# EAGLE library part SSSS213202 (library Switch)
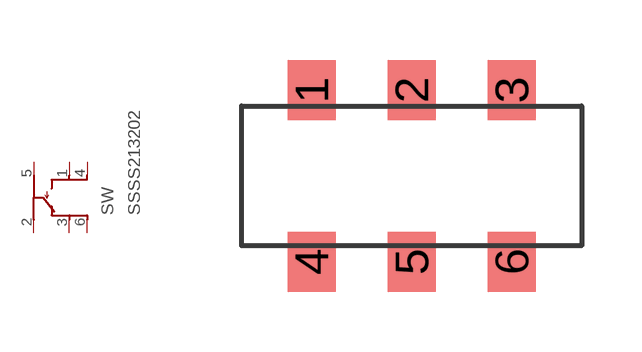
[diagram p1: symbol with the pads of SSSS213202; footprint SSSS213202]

Designator prefix SW

## SSSS213202  [SSSS213202]
1  L1  pas
2  C1  pas
3  R1  pas
4  L2  pas
5  C2  pas
6  R2  pas

## Footprint SSSS213202 (pad centres in mm)
smd 1.2 x 1.5: 1 -2.45,2.2; 2 0.05,2.2; 3 2.55,2.2; 4 -2.45,-2.1; 5 0.05,-2.1; 6 2.55,-2.1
